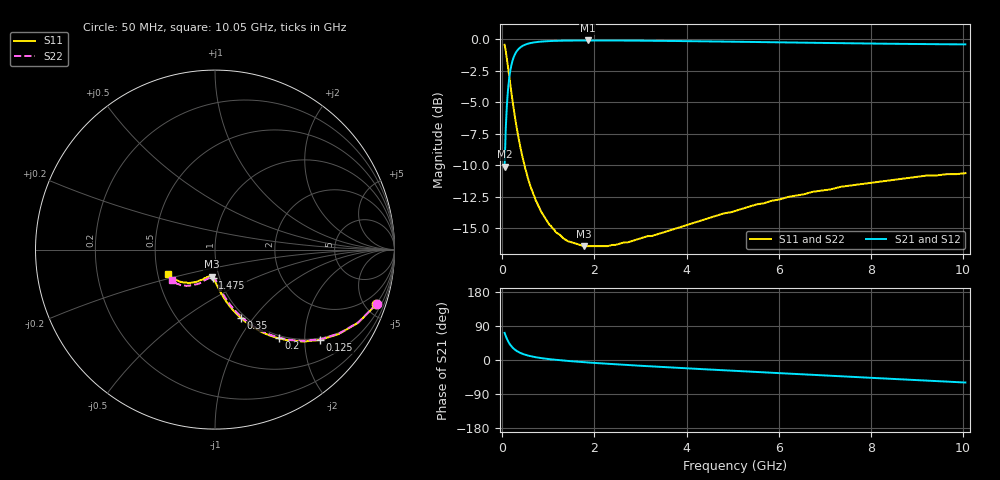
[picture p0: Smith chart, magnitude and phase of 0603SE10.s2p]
! AVX Thin Film Operation		Date: August 2001
! Description: Accu-P® Series, Thin Film, SMD, RF Capacitor
! Part Number: 06035J100FBT
! 50 MHz  -  10.05 GHz
! Serial Measurements
# mhz S db R 50
!	S11		S21		S12		S22
!	dB	Phase	dB	Phase	dB	Phase	dB	Phase
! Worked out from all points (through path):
!   401 points, 50 MHz to 10.05 GHz, reference 50 ohm
!   highest |S21| = -0.11 dB at 1.85 GHz (marker M1); lowest = -10.1 dB at 50 MHz (marker M2)
!   group delay of S21, straight-line fit = 20.8 ps
!   lowest |S11| = -16.4 dB at 1.775 GHz (marker M3), VSWR 1.36, Z = 46 - j14.2 ohm
!   |S11| at or under -10 dB: 482.3 MHz to end of sweep
!   |S22| runs from -16.4 to -0.4 dB; largest |S21 - S12| = 0
!   S11 on the Smith chart (normalised r, x): 50 MHz: 0.95, -5.92; 125 MHz: 0.95, -2.37; 200 MHz: 0.95, -1.49; 350 MHz: 0.95, -0.87; 1.475 GHz: 0.93, -0.30; 10.05 GHz: 0.57, -0.17
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50  -0.45 -18.7  -10.10 71.4  -10.10 71.4  -0.45 -18.6
75  -0.95 -27.0  -7.08 63.1  -7.08 63.1  -0.95 -26.8
125  -2.24 -40.6  -3.95 49.6  -3.95 49.6  -2.24 -40.2
150  -2.95 -46.0  -3.08 44.2  -3.08 44.2  -2.95 -45.5
200  -4.32 -54.4  -2.02 35.9  -2.02 35.9  -4.31 -53.8
275  -6.19 -63.2  -1.20 27.1  -1.20 27.1  -6.19 -62.4
350  -7.78 -69.2  -0.80 21.2  -0.80 21.2  -7.78 -68.2
425  -9.13 -73.6  -0.57 17.0  -0.57 17.0  -9.13 -72.4
525  -10.57 -77.8  -0.40 12.9  -0.40 12.9  -10.57 -76.3
625  -11.81 -81.0  -0.30 9.8  -0.30 9.8  -11.81 -79.2
800  -13.32 -85.1  -0.21 5.9  -0.21 5.9  -13.32 -83.0
1125  -15.09 -90.2  -0.14 0.9  -0.14 0.9  -15.09 -87.5
1475  -16.06 -94.3  -0.12 -3.1  -0.12 -3.1  -16.06 -91.2
1725  -16.35 -96.8  -0.11 -5.4  -0.11 -5.4  -16.35 -93.5
1775  -16.40 -97.2  -0.11 -5.8  -0.11 -5.8  -16.40 -93.8
1850  -16.40 -97.9  -0.11 -6.5  -0.11 -6.5  -16.40 -94.4
2475  -16.28 -103.2  -0.11 -11.4  -0.11 -11.4  -16.28 -99.2
3400  -15.42 -109.9  -0.14 -18.0  -0.14 -18.0  -15.32 -105.8
5050  -13.62 -120.4  -0.21 -28.7  -0.21 -28.7  -13.56 -115.4
6725  -12.10 -132.0  -0.29 -39.0  -0.29 -39.0  -12.10 -126.0
8400  -11.19 -142.2  -0.37 -49.4  -0.37 -49.4  -11.09 -136.1
10050  -10.62 -152.8  -0.42 -59.5  -0.42 -59.5  -10.60 -144.8
